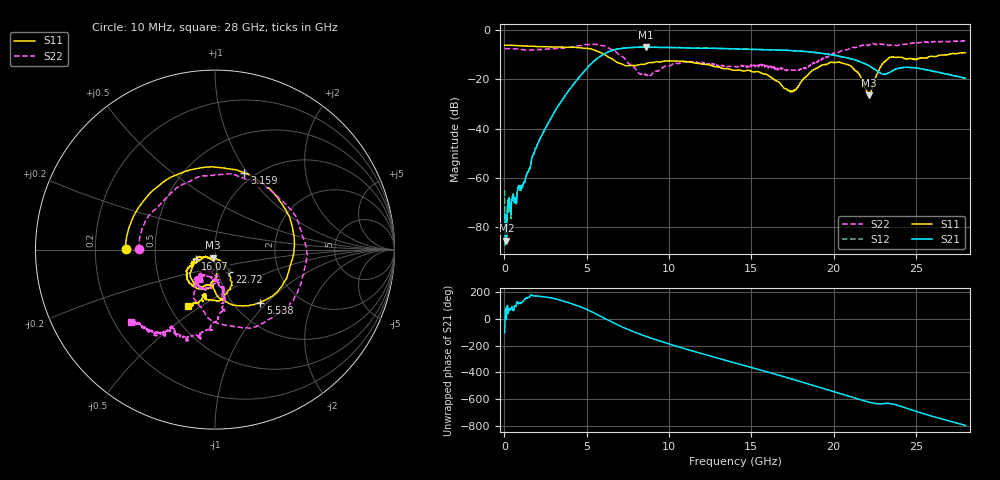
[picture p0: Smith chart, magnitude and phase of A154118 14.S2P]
!  2-Port S-parameters saved by WinCal
! VAR MeasName=S-Parameters (CALIBRATED_DATA) read from VNA (N5230A)
! VAR MeasDate=2015-9-10 14:35:25
! VAR NAME=A154118 14
! VAR FILENAME=A154118 14.S2P
! VAR DATE=2015-9-10 14:35:25
! VAR PHYS_PORTS=1,2
# Hz S DB R 50
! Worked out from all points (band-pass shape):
!   801 points, 10 MHz to 28 GHz, reference 50 ohm
!   highest |S21| = -6.87 dB at 8.582 GHz (marker M1); lowest = -85.6 dB at 115 MHz (marker M2)
!   |S21| within 3 dB of the highest: 5.989 GHz to 19.76 GHz (13.78 GHz wide, 107 % of centre)
!   lowest |S11| = -26.5 dB at 22.12 GHz (marker M3), VSWR 1.10, Z = 48.7 - j4.46 ohm
!   |S11| at or under -10 dB: 6.103 GHz to 26.7 GHz (20.59 GHz wide, 126 % of centre); 26.71534 GHz to 26.79699 GHz (81.65 MHz wide, 0.305 % of centre); 26.82112 GHz to 26.85672 GHz (35.6 MHz wide, 0.133 % of centre)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
!   |S22| runs from -18.8 to -4.1 dB; largest |S21 - S12| = 0.0073
!   S11 on the Smith chart (normalised r, x): 10 MHz: 0.34, +0.00; 3.159 GHz: 0.89, +0.97; 5.538 GHz: 1.32, -0.92; 16.07 GHz: 0.80, -0.08; 22.72 GHz: 1.13, -0.29; 28 GHz: 0.61, -0.44
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1e7  -6.10 179.5  -74.50 -103.3  -65.08 179.7  -7.49 179.8
1.149625e8  -6.05 176.2  -85.62 -4.0  -74.74 72.9  -7.43 176.5
1.1296e9  -6.37 143.1  -63.06 132.8  -62.79 135.2  -7.92 146.1
2.004288e9  -6.61 114.2  -46.41 172.6  -46.49 173.2  -7.85 122.3
3.158875e9  -6.78 69.1  -31.79 148.5  -31.77 148.9  -7.39 81.3
4.698325e9  -7.20 -5.6  -17.88 86.9  -17.83 86.8  -6.16 11.5
5.538025e9  -8.21 -49.4  -12.00 39.2  -11.97 39.1  -5.76 -35.4
6.692612e9  -12.43 -89.2  -7.92 -33.4  -7.91 -33.5  -8.36 -95.9
7.602288e9  -14.38 -92.0  -7.08 -83.7  -7.05 -83.9  -13.90 -124.0
8.581938e9  -13.64 -96.6  -6.87 -129.7  -6.83 -129.9  -17.86 -103.4
9.351662e9  -12.87 -107.4  -6.99 -161.9  -6.95 -162.3  -16.66 -87.7
1.173081e10  -13.39 -138.1  -7.31 109.4  -7.28 108.8  -13.22 -115.6
1.4005e10  -16.26 -146.4  -7.59 30.4  -7.58 29.9  -14.79 -119.6
1.606926e10  -18.54 -154.6  -7.97 -40.6  -7.96 -41.3  -14.78 -122.3
1.746876e10  -24.67 -113.4  -8.28 -90.4  -8.32 -91.1  -16.28 -106.0
1.869332e10  -16.33 -86.6  -8.91 -135.6  -8.93 -136.1  -13.34 -80.5
2.089754e10  -14.12 -135.0  -11.33 141.9  -11.33 141.3  -7.67 -91.4
2.21221e10  -26.53 -104.1  -14.35 96.9  -14.37 96.5  -6.00 -104.5
2.271689e10  -16.52 -57.7  -16.92 83.6  -16.93 83.6  -5.60 -111.9
2.334666e10  -11.26 -79.0  -17.29 86.7  -17.26 86.4  -6.15 -118.1
2.527098e10  -11.17 -102.6  -15.67 16.4  -15.64 15.7  -4.90 -125.2
2.8e10  -9.14 -116.0  -19.49 -78.4  -19.53 -78.5  -4.14 -139.3
